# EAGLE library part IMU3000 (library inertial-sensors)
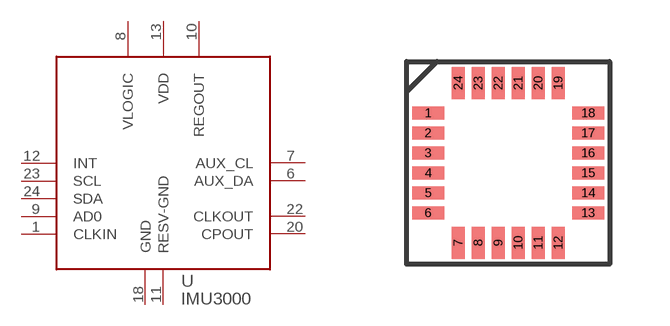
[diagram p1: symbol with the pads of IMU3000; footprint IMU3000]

Designator prefix U

## IMU3000  [IMU3000]
1  CLKIN
6  AUX_DA
7  AUX_CL
8  VLOGIC
9  AD0
10  REGOUT
11  RESV-GND
12  INT
13  VDD
18  GND
20  CPOUT
22  CLKOUT
23  SCL
24  SDA

## Footprint IMU3000 (pad centres in mm)
smd 0.8 x 0.33: 1 -2,1.25; 2 -2,0.75; 3 -2,0.25; 4 -2,-0.25; 5 -2,-0.75; 6 -2,-1.25; 13 2,-1.25; 14 2,-0.75; 15 2,-0.25; 16 2,0.25; 17 2,0.75; 18 2,1.25
smd 0.33 x 0.8: 7 -1.25,-2; 8 -0.75,-2; 9 -0.25,-2; 10 0.25,-2; 11 0.75,-2; 12 1.25,-2; 19 1.25,2; 20 0.75,2; 21 0.25,2; 22 -0.25,2; 23 -0.75,2; 24 -1.25,2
